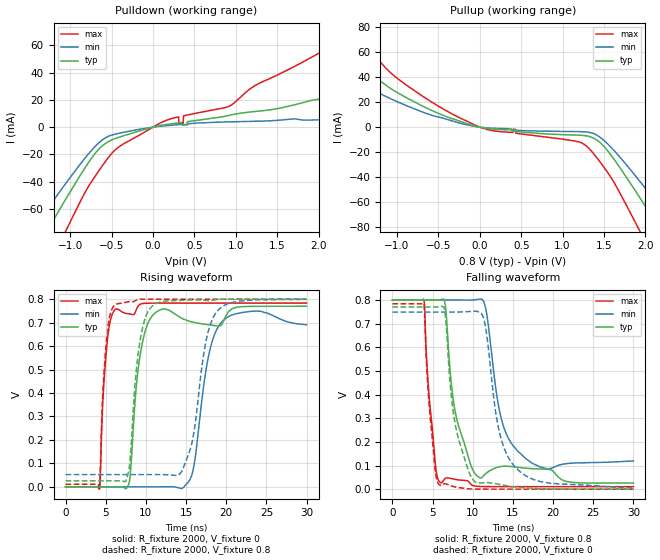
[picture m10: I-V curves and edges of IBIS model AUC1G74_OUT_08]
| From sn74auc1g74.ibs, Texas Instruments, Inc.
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[Model]   AUC1G74_OUT_08
Model_type  Output
Vref =   0
Rref =   2000
Cref =   15p
Vmeas =   0.4
| variable   typ   min   max
C_comp   5.95pF   2.12pF   7.79pF
| C_pullup   5.73pF   2.12pF   7.79pF
| C_pulldown   6.17pF   5.32pF   6.79pF
[Temperature Range]   40   100   -40
| Ambient temperature   25   85   -40
[Voltage range]   0.8   0.8   0.8
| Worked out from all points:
|   slope of the pulldown table from 0 to 0.12 V, typ, clamps not added: 76.8 ohm
|   slope of the pullup table from 0 to 0.12 V, typ, clamps not added: 93 ohm
|   rising waveform, R_fixture 2000, V_fixture 0: 20-80 % time 1.31ns typ, 1.58ns min, 794ps max; typ from 0 V to 0.77 V
|   falling waveform, R_fixture 2000, V_fixture 0.8: 20-80 % time 2.18ns typ, 1.89ns min, 1.05ns max; typ from 0.8 V to 0.026 V
|   rising waveform, R_fixture 2000, V_fixture 0.8: 20-80 % time 1.21ns typ, 1.85ns min, 731ps max; typ from 0.025 V to 0.8 V
|   falling waveform, R_fixture 2000, V_fixture 0: 20-80 % time 1.91ns typ, 2.22ns min, 986ps max; typ from 0.77 V to 0 V
[Pulldown]
| AUC1G74_OUT_08
|   Voltage   I(typ)   I(min)   I(max)
-3.6V     -318.5mA   -267.5mA   -388.7mA
-1.505V   -99.39mA   -79.75mA   -132.3mA
-1.265V   -74.51mA   -59.06mA   -102.6mA
-1.06V    -53.52mA   -41.83mA   -77.02mA
-680mV    -17.89mA   -13.04mA   -34.39mA
-355mV    -6.313mA   -3.814mA   -12.25mA
920mV     8.612mA    3.848mA    15.28mA
2.655V    17.26mA    6.103mA    74.33mA
3.075V    18.7mA     6.623mA    73.96mA
3.43V     19.91mA    7.073mA    61.16mA
5.055V    25.59mA    9.257mA    74.88mA
7.2V      33.99mA    12.46mA    100.5mA
[Pullup]
| AUC1G74_OUT_08
|   Voltage   I(typ)   I(min)   I(max)
-3.6V     150.2mA    25.75mA    270.7mA
-1.915V   81.31mA    24.24mA    112.5mA
-1.565V   57.79mA    31.39mA    81.74mA
-1.025V   28.72mA    21.13mA    40.41mA
-225mV    4.374mA    2.948mA    6.84mA
1.255V    -6.674mA   -3.704mA   -13.49mA
1.515V    -16.55mA   -11.53mA   -33.48mA
1.865V    -49.44mA   -37.64mA   -74.32mA
1.98V     -61.14mA   -47.13mA   -88.92mA
2.105V    -74.02mA   -57.66mA   -104.8mA
2.39V     -103.8mA   -82.23mA   -140.9mA
7.2V      -610.8mA   -518.6mA   -738.2mA
[Ramp]
| AUC1G74_OUT_08
| variable   typ   min   max
dV/dt_r   0.47/1.31E-09   0.45/1.86E-09   0.48/7.94E-10
dV/dt_f   0.47/2.18E-09   0.43/2.18E-09   0.48/1.05E-09
R_load = 2000
[Rising Waveform]
| AUC1G74_OUT_08
R_fixture =   2000
C_fixture =   0
L_fixture =   0
V_fixture =   0
V_fixture_min = 0
V_fixture_max = 0
|   Time   V(typ)   V(min)   V(max)
0s        9.41nV     53.68nV    554pV
4.255ns   -149.1nV   275.2nV    -7.533mV
5.04ns    -1.854uV   68.19nV    566.2mV
6.18ns    -10.4uV    -49.08nV   756.7mV
7.92ns    18.85mV    -1.103uV   737.4mV
9.205ns   545.1mV    -4.445uV   776.8mV
11ns      737.3mV    -3.47uV    783.4mV
15.59ns   704.6mV    38.5mV     783.7mV
19.51ns   696.3mV    705.9mV    783.7mV
29.99ns   769.9mV    690.8mV    783.7mV
[Falling Waveform]
| AUC1G74_OUT_08
R_fixture =   2000
C_fixture =   0
L_fixture =   0
V_fixture =   0.8
V_fixture_min = 0.8
V_fixture_max = 0.8
|   Time   V(typ)   V(min)   V(max)
0s        800mV      800mV      800mV
3.93ns    800mV      800mV      797.4mV
4.605ns   800mV      800mV      376mV
5.915ns   800mV      800mV      29.26mV
6.565ns   780.5mV    800mV      44.94mV
7.9ns     312mV      799.8mV    40.82mV
10.51ns   57.03mV    801.8mV    12.17mV
13.61ns   96.37mV    290mV      10.73mV
15.58ns   92.5mV     161.6mV    10.68mV
29.99ns   25.66mV    119.4mV    10.62mV
[Rising Waveform]
| AUC1G74_OUT_08
R_fixture =   2000
C_fixture =   0
L_fixture =   0
V_fixture =   0.8
V_fixture_min = 0.8
V_fixture_max = 0.8
|   Time   V(typ)   V(min)   V(max)
0s        25.46mV    52.07mV    10.6mV
4.23ns    25.46mV    52.07mV    9.28mV
5.04ns    25.46mV    52.07mV    607.4mV
6.14ns    25.48mV    52.07mV    776.3mV
7.855ns   66.59mV    52.07mV    789.3mV
9.12ns    588.5mV    52.08mV    799.5mV
10.73ns   769.2mV    52.13mV    799.9mV
14.62ns   795.7mV    77.67mV    799.9mV
18.96ns   799.4mV    752.5mV    799.9mV
29.99ns   799.9mV    799.5mV    800mV
[Falling Waveform]
| AUC1G74_OUT_08
R_fixture =   2000
C_fixture =   0
L_fixture =   0
V_fixture =   0
V_fixture_min = 0
V_fixture_max = 0
|   Time   V(typ)   V(min)   V(max)
0s        770mV      748.6mV    783.8mV
3.915ns   770mV      748.6mV    781.5mV
4.62ns    770mV      748.6mV    335.3mV
5.83ns    770.9mV    748.6mV    18.7mV
6.535ns   749.2mV    748.6mV    22.91mV
7.89ns    261.5mV    748.7mV    8.599mV
10.23ns   32.68mV    752.1mV    441.8uV
11.4ns    27.47mV    716.9mV    190uV
15.26ns   8.9mV      93.96mV    74.75uV
29.99ns   102.9uV    4.917mV    24.31uV
